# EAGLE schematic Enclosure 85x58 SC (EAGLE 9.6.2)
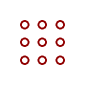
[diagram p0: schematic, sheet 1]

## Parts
U$1  PROTO-28X18-SUPPORT  [PROTO-28X18-SUPPORT]

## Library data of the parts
U$1 = digitalconcepts:PROTO-28X18-SUPPORT: 28 x 18 Prototyping board to fit an 85 x 58 enclosure, with external connector cut-outs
